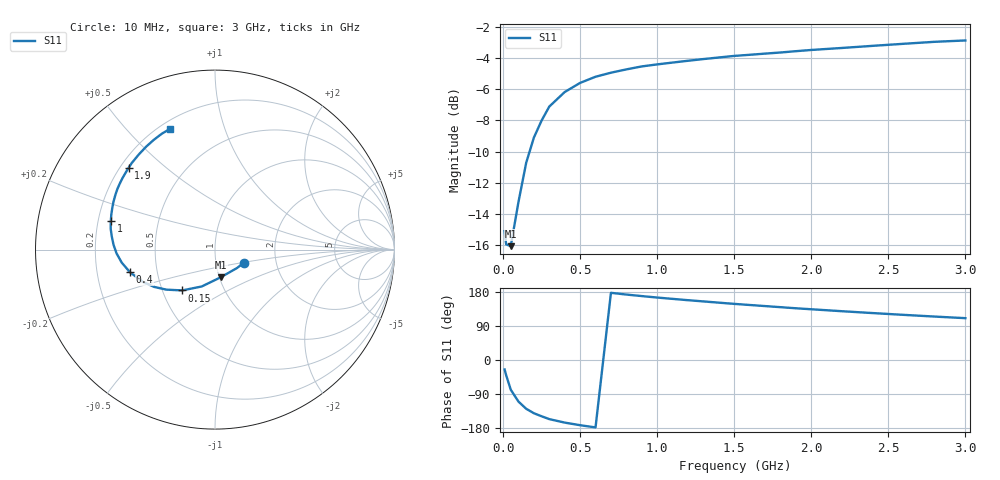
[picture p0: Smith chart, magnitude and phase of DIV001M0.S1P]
! SIEMENS Small Signal Semiconductors
! BAV99
! Silicon Switching Diode in SOT23
! IF = 1 mA
! S-Parameters:  May  1995
# GHz  S  MA  R  50
!  f  S11
! GHz  MAG  ANG
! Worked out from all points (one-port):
!   30 points, 10 MHz to 3 GHz, reference 50 ohm
!   lowest |S11| = -16.0 dB at 50 MHz (marker M1), VSWR 1.37, Z = 50.7 - j16.1 ohm
!   |S11| at or under -10 dB: start of sweep to 172.1 MHz
!   S11 on the Smith chart (normalised r, x): 10 MHz: 1.36, -0.21; 150 MHz: 0.63, -0.31; 400 MHz: 0.35, -0.11; 1 GHz: 0.25, +0.13; 1.9 GHz: 0.23, +0.38; 3 GHz: 0.24, +0.67
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0.01  0.1761 -25.0
0.02  0.1597 -40.1
0.05  0.1576 -78.5
0.1  0.2184 -109.8
0.15  0.2913 -128.7
0.2  0.3508 -140.5
0.25  0.3977 -148.5
0.3  0.4409 -156.0
0.4  0.4908 -165.2
0.5  0.5249 -172.1
0.6  0.5492 -177.9
0.7  0.5659 177.3
0.8  0.5799 172.7
0.9  0.5927 168.7
1  0.6016 164.8
1.2  0.6179 157.8
1.3  0.6257 154.6
1.4  0.6331 151.3
1.5  0.6404 148.1
1.6  0.6457 145.2
1.7  0.6514 142.3
1.9  0.6631 136.5
2  0.6691 133.9
2.2  0.6791 128.7
2.4  0.6898 123.8
2.6  0.7003 119.1
2.8  0.7106 114.6
3  0.7177 110.4
